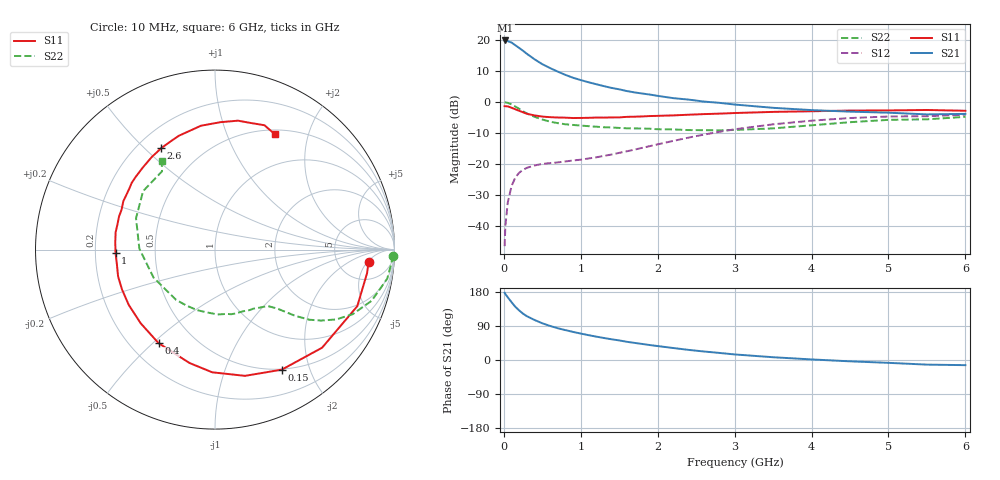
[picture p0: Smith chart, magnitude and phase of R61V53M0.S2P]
! SIEMENS Small Signal Semiconductors
! BFR193
! Si NPN RF Bipolar Junction Transistor in SOT23
! VCE = 1.5 V  IC = 3 mA
! Common Emitter S-Parameters:  May  1996
# GHz  S  MA  R  50
!  f  S11  S21  S12  S22
! GHz  MAG  ANG  MAG  ANG  MAG  ANG  MAG  ANG
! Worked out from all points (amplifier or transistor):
!   36 points, 10 MHz to 6 GHz, reference 50 ohm
!   highest |S21| = 19.9 dB at 20 MHz (marker M1)
!   |S21| within 3 dB of that: start of sweep to 231.1 MHz
!   unconditionally stable (mu >= 1): 1.03 GHz to 2.09 GHz
!   at 250 MHz: K = 0.31, MSG = 19.2 dB, |S12| = -21.9 dB
!   at 1.4 GHz: K = 1.10, MAG = 8.8 dB, |S12| = -16.9 dB
!   at 6 GHz: K = 0.99, MSG = 0.1 dB, |S12| = -4.1 dB
!   S11 on the Smith chart (normalised r, x): 10 MHz: 10, -5; 150 MHz: 0.49, -1.59; 400 MHz: 0.31, -0.52; 1 GHz: 0.29, -0.01; 2.6 GHz: 0.29, +0.56; 6 GHz: 0.55, +1.50
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0.01  0.8589 -4.5  9.897 177.4  0.0047 88.7  0.9948 -1.9
0.02  0.8572 -8.9  9.904 174.0  0.0099 85.8  0.987 -3.9
0.05  0.8531 -21.7  9.665 165.8  0.0236 78.6  0.9732 -9.6
0.1  0.8092 -42.5  9.157 152.6  0.0439 68.4  0.918 -18.1
0.15  0.7654 -60.9  8.276 140.2  0.0607 59.8  0.8468 -25.2
0.2  0.7231 -76.6  7.483 130.7  0.0723 53.2  0.7785 -30.0
0.25  0.6838 -91.3  6.74 122.2  0.0807 48.1  0.7106 -33.8
0.3  0.6475 -102.7  6.021 115.5  0.0867 44.9  0.6555 -36.6
0.4  0.6087 -121.1  4.906 105.5  0.0947 40.1  0.5782 -39.6
0.5  0.583 -135.3  4.097 96.9  0.1004 38.2  0.5235 -41.5
0.6  0.5709 -147.3  3.549 89.9  0.1033 37.8  0.4831 -43.2
0.7  0.5637 -156.7  3.112 83.9  0.106 38.3  0.4574 -44.8
0.8  0.5603 -164.5  2.752 78.9  0.1099 39.5  0.438 -46.3
1  0.5545 -178.2  2.266 69.7  0.1174 42.9  0.4176 -49.8
1.1  0.5572 175.9  2.093 65.6  0.1226 45.1  0.4085 -52.3
1.6  0.5775 152.2  1.506 48.0  0.1605 54.6  0.3772 -65.8
2.2  0.6095 131.1  1.159 31.7  0.2356 57.3  0.3619 -87.6
2.6  0.6395 117.9  1.02 22.5  0.2983 54.3  0.3518 -106.2
3.5  0.6945 96.5  0.808 7.3  0.4372 40.2  0.3762 -155.5
4.5  0.7296 79.9  0.701 -3.5  0.5524 21.6  0.4735 158.3
5.5  0.7456 68.3  0.633 -12.2  0.5908 3.8  0.5265 124.1
6  0.7243 62.7  0.645 -13.6  0.6253 -1.2  0.578 120.9
